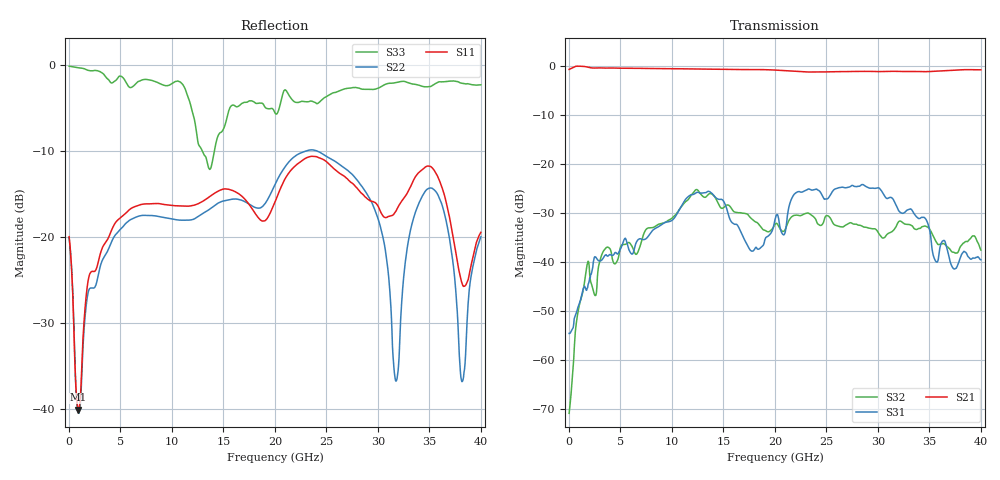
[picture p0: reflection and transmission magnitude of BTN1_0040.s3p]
! MARKI MICROWAVE INC.
! Email:  info@markimicrowave.com  Phone:  408-778-4200
! Model Number:  BTN1-0040  Date:  06/13
! Filename:		BTN1_0040.S3P  Version: 1.0
! Description:  3-port S-parameter data for Bias Tee BTN1-0040
! Frequency Range: 	10 MHz to 40 GHz
! Port Configuration:	PORT 1: RF & DC
!  PORT 2: RF
!  Port 3: DC
! S3P File: Measurements: Mag<S11> Ang<S11> Mag<S12> Ang<S12> Mag<S13> Ang<S13> ! row 1
!  Mag<S21> Ang<S21> Mag<S22> Ang<S22> Mag<S23> Ang<S23> ! row 2
!  Mag<S31> Ang<S31> Mag<S32> Ang<S32> Mag<S33> Ang<S33> ! row 3
# GHz S  dB  R 50
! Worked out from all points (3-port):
!   801 points, 10 MHz to 40 GHz, reference 50 ohm
!   strongest paths, dB at 10 MHz, 10.01 GHz, 20.01 GHz, 30.01 GHz, 40 GHz:
!     S21: -0.7, -0.6, -0.9, -1.2, -0.8
!     S31: -54.6, -31.6, -31.4, -24.9, -39.6
!     S32: -70.9, -31.1, -32.4, -34.0, -37.6
!   lowest |S11| = -40.1 dB at 910 MHz (marker M1), VSWR 1.02, Z = 50.9 - j0.484 ohm
!   |S11| at or under -10 dB: start of sweep to end of sweep
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0.01  -20.00 144.2  -0.77 1.0  -53.33 66.0
      -0.75 0.9  -20.11 142.9  -62.08 -101.4
      -54.64 56.7  -70.95 113.3  -0.18 172.2
0.91  -40.10 -28.8  -0.09 -19.6  -48.91 21.0
      -0.09 -19.6  -40.50 -22.4  -49.52 -110.3
      -49.08 21.2  -49.80 -109.4  -0.37 117.9
4.01  -19.61 168.9  -0.45 -87.8  -38.51 -113.1
      -0.46 -87.8  -20.93 -173.8  -37.40 65.8
      -38.57 -113.0  -37.47 66.1  -2.04 -81.2
7.96  -16.18 77.5  -0.55 -173.3  -33.99 88.9
      -0.56 -173.3  -17.54 105.8  -33.05 -85.5
      -34.00 88.7  -33.08 -85.5  -1.81 36.4
12.86  -15.97 -45.6  -0.67 80.4  -25.99 -159.6
       -0.68 80.3  -17.39 33.3  -26.37 26.2
       -26.01 -159.6  -26.37 26.2  -9.82 107.1
20.01  -15.94 66.6  -0.87 -75.6  -31.31 -79.0
       -0.89 -75.7  -13.92 -30.9  -32.38 67.5
       -31.38 -78.8  -32.39 67.7  -5.63 69.4
28.91  -15.52 -126.4  -1.13 93.1  -24.73 178.5
       -1.15 93.0  -14.98 177.5  -33.08 4.1
       -24.74 178.6  -33.00 3.9  -2.87 -82.1
32.11  -16.22 -119.9  -1.15 23.2  -29.76 8.5
       -1.17 23.1  -32.41 -79.2  -31.69 -142.2
       -29.83 7.8  -31.71 -142.2  -2.00 96.4
37.51  -21.44 142.9  -0.87 -94.4  -41.31 150.5
       -0.87 -94.5  -25.52 -171.8  -38.33 -66.0
       -41.41 151.8  -38.25 -67.7  -1.92 177.5
40  -19.49 -32.1  -0.83 -150.9  -39.63 60.7
    -0.84 -151.1  -20.01 -39.7  -37.59 141.5
    -39.60 59.3  -37.63 143.3  -2.35 37.9
